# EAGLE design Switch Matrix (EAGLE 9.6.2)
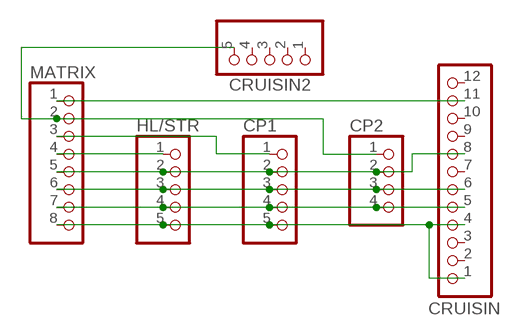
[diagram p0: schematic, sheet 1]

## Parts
CP1  PINHD-1X5  [1X05]
CP2  PINHD-1X4  [1X04]
CRUISIN  PINHD-1X12  [1X12]
CRUISIN2  PINHD-1X5  [1X05]
HL/STR  PINHD-1X5  [1X05]
MATRIX  PINHD-1X8  [1X08]

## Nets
N$1: CP2.1 CRUISIN2.5 MATRIX.2
N$3: CP1.4 CP2.4 CRUISIN.5 HL/STR.4 MATRIX.7
N$4: CP1.3 CP2.3 CRUISIN.6 HL/STR.3 MATRIX.6
N$5: CP1.2 CP2.2 CRUISIN.8 HL/STR.2 MATRIX.5
N$6: HL/STR.1 MATRIX.4
N$7: CP1.1 MATRIX.3
N$8: CP1.5 CRUISIN.1 CRUISIN.4 HL/STR.5 MATRIX.8
N$9: CRUISIN.11 MATRIX.1
Unconnected: CRUISIN2.1 CRUISIN2.2 CRUISIN2.3 CRUISIN2.4 CRUISIN.2 CRUISIN.3 CRUISIN.7 CRUISIN.9 CRUISIN.10 CRUISIN.12

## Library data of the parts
CP1 CRUISIN2 HL/STR = pinhead:PINHD-1X5: PIN HEADER
CP2 = pinhead:PINHD-1X4: PIN HEADER
CRUISIN = pinhead:PINHD-1X12: PIN HEADER
MATRIX = pinhead:PINHD-1X8: PIN HEADER

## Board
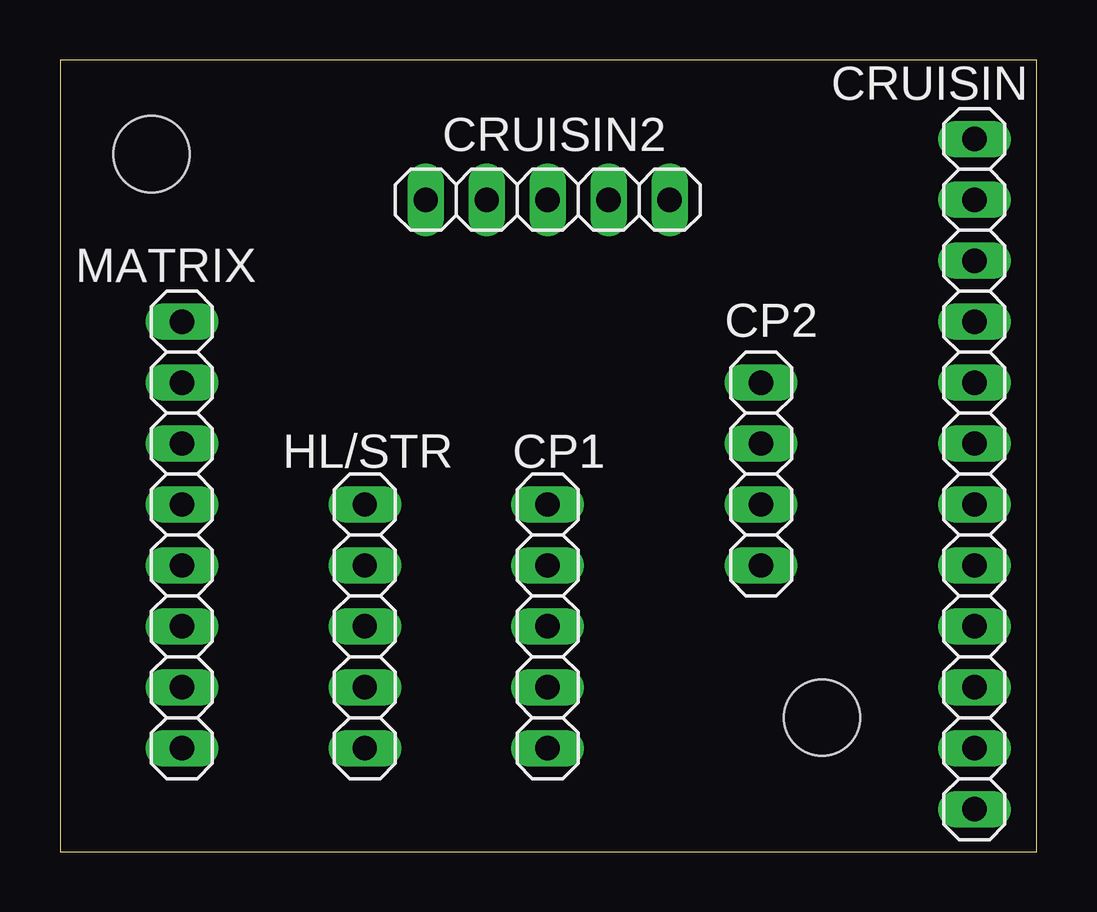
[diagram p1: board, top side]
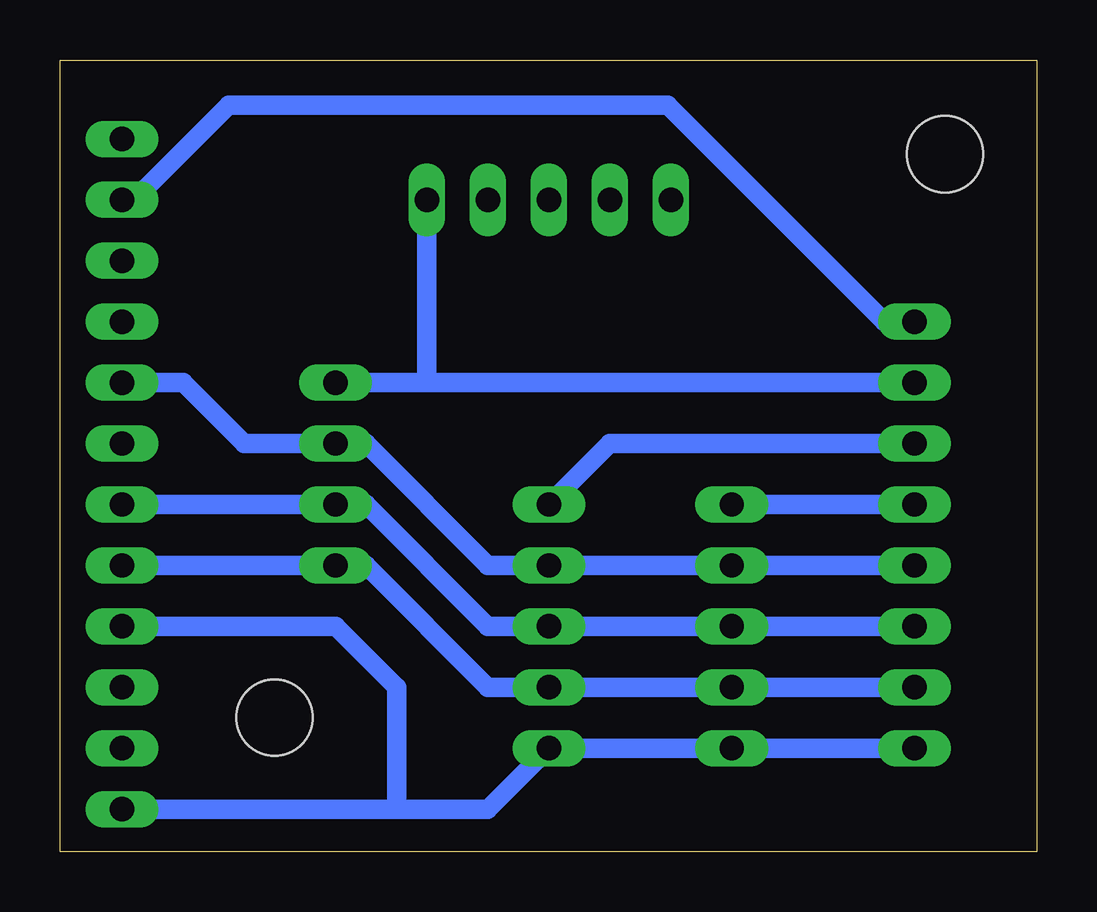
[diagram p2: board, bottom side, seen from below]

Size 40.69 x 33.01 mm. Coordinates in mm from the lower left corner, seen from the top.
Outline: 0,0 40.69,0 40.69,33.01 0,33.01 0,0
Copper layers (1*16): Top 0.035mm / dielectric 1.5mm / Bottom 0.035mm
Design rules "default": minimum track width 6mil, minimum drill 0.35mm, track to track 6mil, track to pad 6mil, pad to pad 6mil, via to via 6mil, smd to smd 6mil, copper to edge 40mil, drill to drill 6mil, minimum pad ring 10mil, minimum via ring 8mil, stop-mask expansion 4mil, vias tented up to drill 0mil, thermal gap 10mil
Holes 3.17 mm at 3.81,29.08 31.75,5.59
tRestrict: area 0.6,25.9 to 7,32.3; area 28.6,2.4 to 34.9,8.8

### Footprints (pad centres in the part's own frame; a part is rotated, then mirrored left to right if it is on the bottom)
1X05 = drill 1.016 long: 1 -5.08,0; 2 -2.54,0; 3 0,0; 4 2.54,0; 5 5.08,0
1X04 = drill 1.016 long: 1 -3.81,0; 2 -1.27,0; 3 1.27,0; 4 3.81,0
1X12 = drill 1.016 long: 1 -13.97,0; 2 -11.43,0; 3 -8.89,0; 4 -6.35,0; 5 -3.81,0; 6 -1.27,0; 7 1.27,0; 8 3.81,0; 9 6.35,0; 10 8.89,0; 11 11.43,0; 12 13.97,0
1X08 = drill 1.016 long: 1 -8.89,0; 2 -6.35,0; 3 -3.81,0; 4 -1.27,0; 5 1.27,0; 6 3.81,0; 7 6.35,0; 8 8.89,0

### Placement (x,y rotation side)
CP1  20.32,9.4 270 top
CP2  29.21,15.75 270 top
CRUISIN  38.1,15.75 90 top
CRUISIN2  20.32,27.18 0 top
HL/STR  12.7,9.4 270 top
MATRIX  5.08,13.21 270 top

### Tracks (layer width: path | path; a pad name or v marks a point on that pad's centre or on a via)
N$1
  Bottom 0.813: CP2.1 25.4,19.56 | 25.4,19.56 MATRIX.2 | CRUISIN2.5 25.4,19.56
N$3
  Bottom 0.813: HL/STR.4 CP1.4 22.86,6.86 27.94,11.94 CP2.4 CRUISIN.5 | 11.43,6.86 HL/STR.4 | HL/STR.4 MATRIX.7
N$4
  Bottom 0.813: CP1.3 22.86,9.4 27.94,14.48 CP2.3 CRUISIN.6 | 19.05,9.4 CP1.3 | CP1.3 HL/STR.3 MATRIX.6
N$5
  Bottom 0.813: MATRIX.5 HL/STR.2 CP1.2 22.86,11.94 27.94,17.02 CP2.2 33.02,17.02 35.56,19.56 CRUISIN.8
N$6
  Bottom 0.813: HL/STR.1 MATRIX.4
N$7
  Bottom 0.813: CP1.1 17.78,17.02 MATRIX.3
N$8
  Bottom 0.813: MATRIX.8 HL/STR.5 CP1.5 22.86,1.78 26.67,1.78 | CRUISIN.1 26.67,1.78 | CRUISIN.4 29.21,9.4 26.67,6.86 26.67,1.78
N$9
  Bottom 0.813: CRUISIN.11 37.59,27.18 33.66,31.11 15.37,31.11 6.35,22.1 MATRIX.1

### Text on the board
Document: Col8 | C8 | C9 | Col9 | C10 | C11 | R0 | R1 | R2 | R3 | Col11 | Col10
